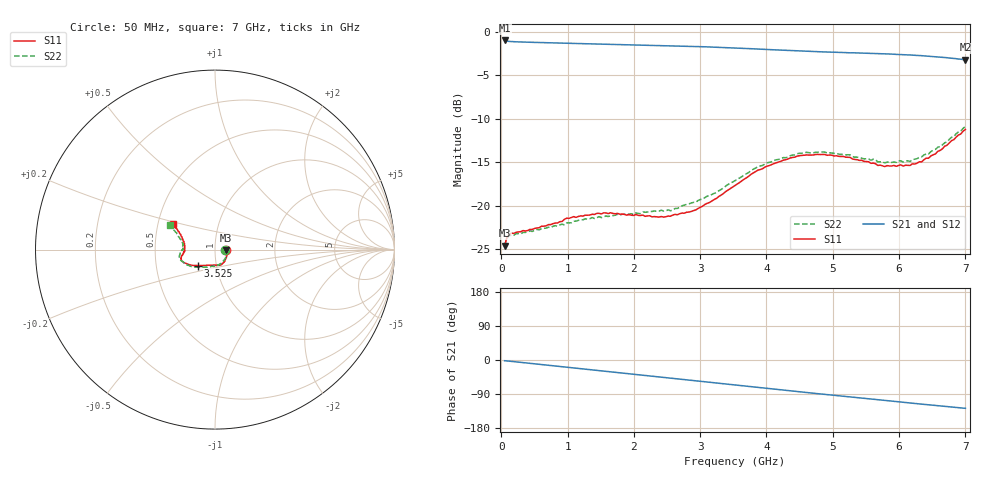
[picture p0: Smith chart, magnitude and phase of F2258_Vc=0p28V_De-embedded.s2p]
! Integrated Device Technology
! Corporate Headquarters
! 6024 Silver Creek Valley Road
! San Jose, CA 95138  USA
! Phone:  1-408-284-8200
! Toll Free:  1-800-223-1366
! Webpage:  http://www.idt.com/
! Timing and RF Division
! 515 Groton Road, Suite 102
! Westford, MA 01886-6024
! Device:  F2258
! Description: Voltage Variable RF Attenuator
! Frequency:  50.0 -  6000.00 MHz
! Package:  3x3 mm Thin QFN Plastic Package: 16 pin
! Ports:  2 RF, 2 DC
!  Pin  1  = NC
!  Pin  2  = NC
!  Pin  3  = RF2  = Port 2
!  Pin  4  = GND
!  Pin  5  = Vdd
!  Pin  6  = NC
!  Pin  7  = VCTRL
!  Pin  8  = NC
!  Pin  9  = GND
!  Pin 10  = RF1  = Port 1
!  Pin 11  = NC
!  Pin 12  = NC
!  Pin 13  = NC
!  Pin 14  = NC
!  Pin 15  = NC
!  Pin 16  = NC
! Vcntrl:  0.280 Volts
! Vdd:  +3.300 Volts
! Current:  1.082 mA
! Data:  The device was measured on a the F2258 evaluation board which has
!  individual transmission lines to the RF pins.  Data was collected
!  using a calibrated network analyzer.  The evaluation board was
!  de-embedded using a TRL calibration technique.
!  The reference plane is the edge of the package pin.
! Misc:  SN 10
!  Action Tracker AT0285
! Date Measured:  2014-12-10
! Date:  2016-01-13  MJV
! Note:
!  Integrated Device Technology supplies this data as a sample of measured
!  data at the package pin for this product.  Your particular data for this
!  product may vary.
!  Data was taken at 25 degrees C.
!  Integrated Device Technology reserves the right to change this data at anytime.
!Freq_(GHz)  S11M_(dB)  S11P_(deg)  S21M_(dB)  S21P_(deg)  S12M_(dB)  S12P_(deg)  S22M_(dB)  S22P_(deg)
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# GHz S dB R 50
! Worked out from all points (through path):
!   201 points, 50 MHz to 7 GHz, reference 50 ohm
!   highest |S21| = -0.97 dB at 50 MHz (marker M1); lowest = -3.2 dB at 7 GHz (marker M2)
!   group delay of S21, straight-line fit = 50.5 ps
!   lowest |S11| = -24.6 dB at 50 MHz (marker M3), VSWR 1.12, Z = 56.2 - j0.397 ohm
!   |S11| at or under -10 dB: start of sweep to end of sweep
!   |S22| runs from -24.7 to -10.9 dB; largest |S21 - S12| = 0.00043
!   S11 on the Smith chart (normalised r, x): 50 MHz: 1.12, -0.01; 3.525 GHz: 0.81, -0.15; 7 GHz: 0.60, +0.19
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0.05  -24.63 -3.4  -0.97 -1.9  -0.97 -1.9  -24.69 -3.0
0.08475  -23.66 -5.8  -1.05 -2.5  -1.05 -2.5  -23.76 -5.4
0.15425  -23.19 -9.1  -1.10 -3.6  -1.10 -3.6  -23.38 -9.3
0.71025  -22.20 -36.5  -1.24 -14.1  -1.23 -14.1  -22.50 -38.2
0.98825  -21.46 -50.2  -1.29 -19.3  -1.29 -19.3  -22.01 -54.2
1.2315  -21.23 -58.5  -1.34 -23.8  -1.34 -23.8  -21.65 -63.2
1.6485  -20.83 -70.1  -1.43 -31.4  -1.43 -31.4  -21.17 -76.2
2.37825  -21.34 -91.3  -1.56 -44.8  -1.56 -44.8  -20.65 -93.9
2.552  -21.24 -97.3  -1.59 -48.0  -1.59 -48.0  -20.61 -99.2
2.93425  -20.50 -114.0  -1.67 -55.1  -1.67 -55.1  -19.62 -112.6
3.247  -19.17 -126.6  -1.75 -61.0  -1.75 -61.0  -18.50 -124.8
3.525  -17.71 -136.9  -1.84 -66.2  -1.83 -66.2  -17.14 -135.3
4.0115  -15.45 -150.8  -2.01 -75.2  -2.01 -75.2  -15.07 -150.8
4.46325  -14.31 -159.2  -2.17 -83.4  -2.18 -83.4  -14.03 -161.9
4.7065  -14.17 -162.5  -2.25 -87.7  -2.25 -87.7  -13.92 -166.1
5.2625  -14.45 -169.4  -2.40 -97.4  -2.40 -97.4  -14.17 -174.2
5.6795  -15.38 -176.2  -2.48 -104.6  -2.48 -104.6  -14.98 -179.6
5.85325  -15.44 179.6  -2.54 -107.8  -2.54 -107.8  -15.01 175.8
6.166  -15.38 171.8  -2.64 -113.4  -2.65 -113.4  -14.92 169.9
6.33975  -14.97 165.4  -2.73 -116.5  -2.73 -116.5  -14.38 165.5
6.722  -13.06 153.7  -2.96 -123.1  -2.96 -123.1  -12.68 156.4
7  -11.23 148.2  -3.20 -127.4  -3.21 -127.4  -10.89 151.5
